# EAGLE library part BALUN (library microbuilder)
BALUN - Baluns for RF 1206 800-1000MHz Balun (1206) - Digikey: 712-1023-1-ND
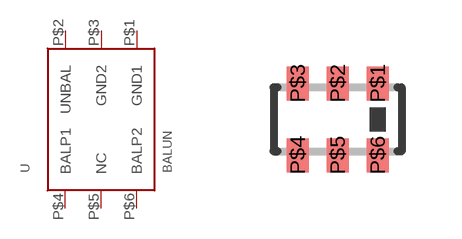
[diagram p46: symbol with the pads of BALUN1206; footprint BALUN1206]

Designator prefix U

## BALUN  [BALUN1206]
P$1  GND1
P$2  UNBAL
P$3  GND2
P$4  BALP1
P$5  NC
P$6  BALP2

## Footprint BALUN1206 (pad centres in mm)
smd 0.55 x 0.85: P$1 1,0.9; P$2 0,0.9; P$3 -1,0.9; P$4 -1,-0.9; P$5 0,-0.9; P$6 1,-0.9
